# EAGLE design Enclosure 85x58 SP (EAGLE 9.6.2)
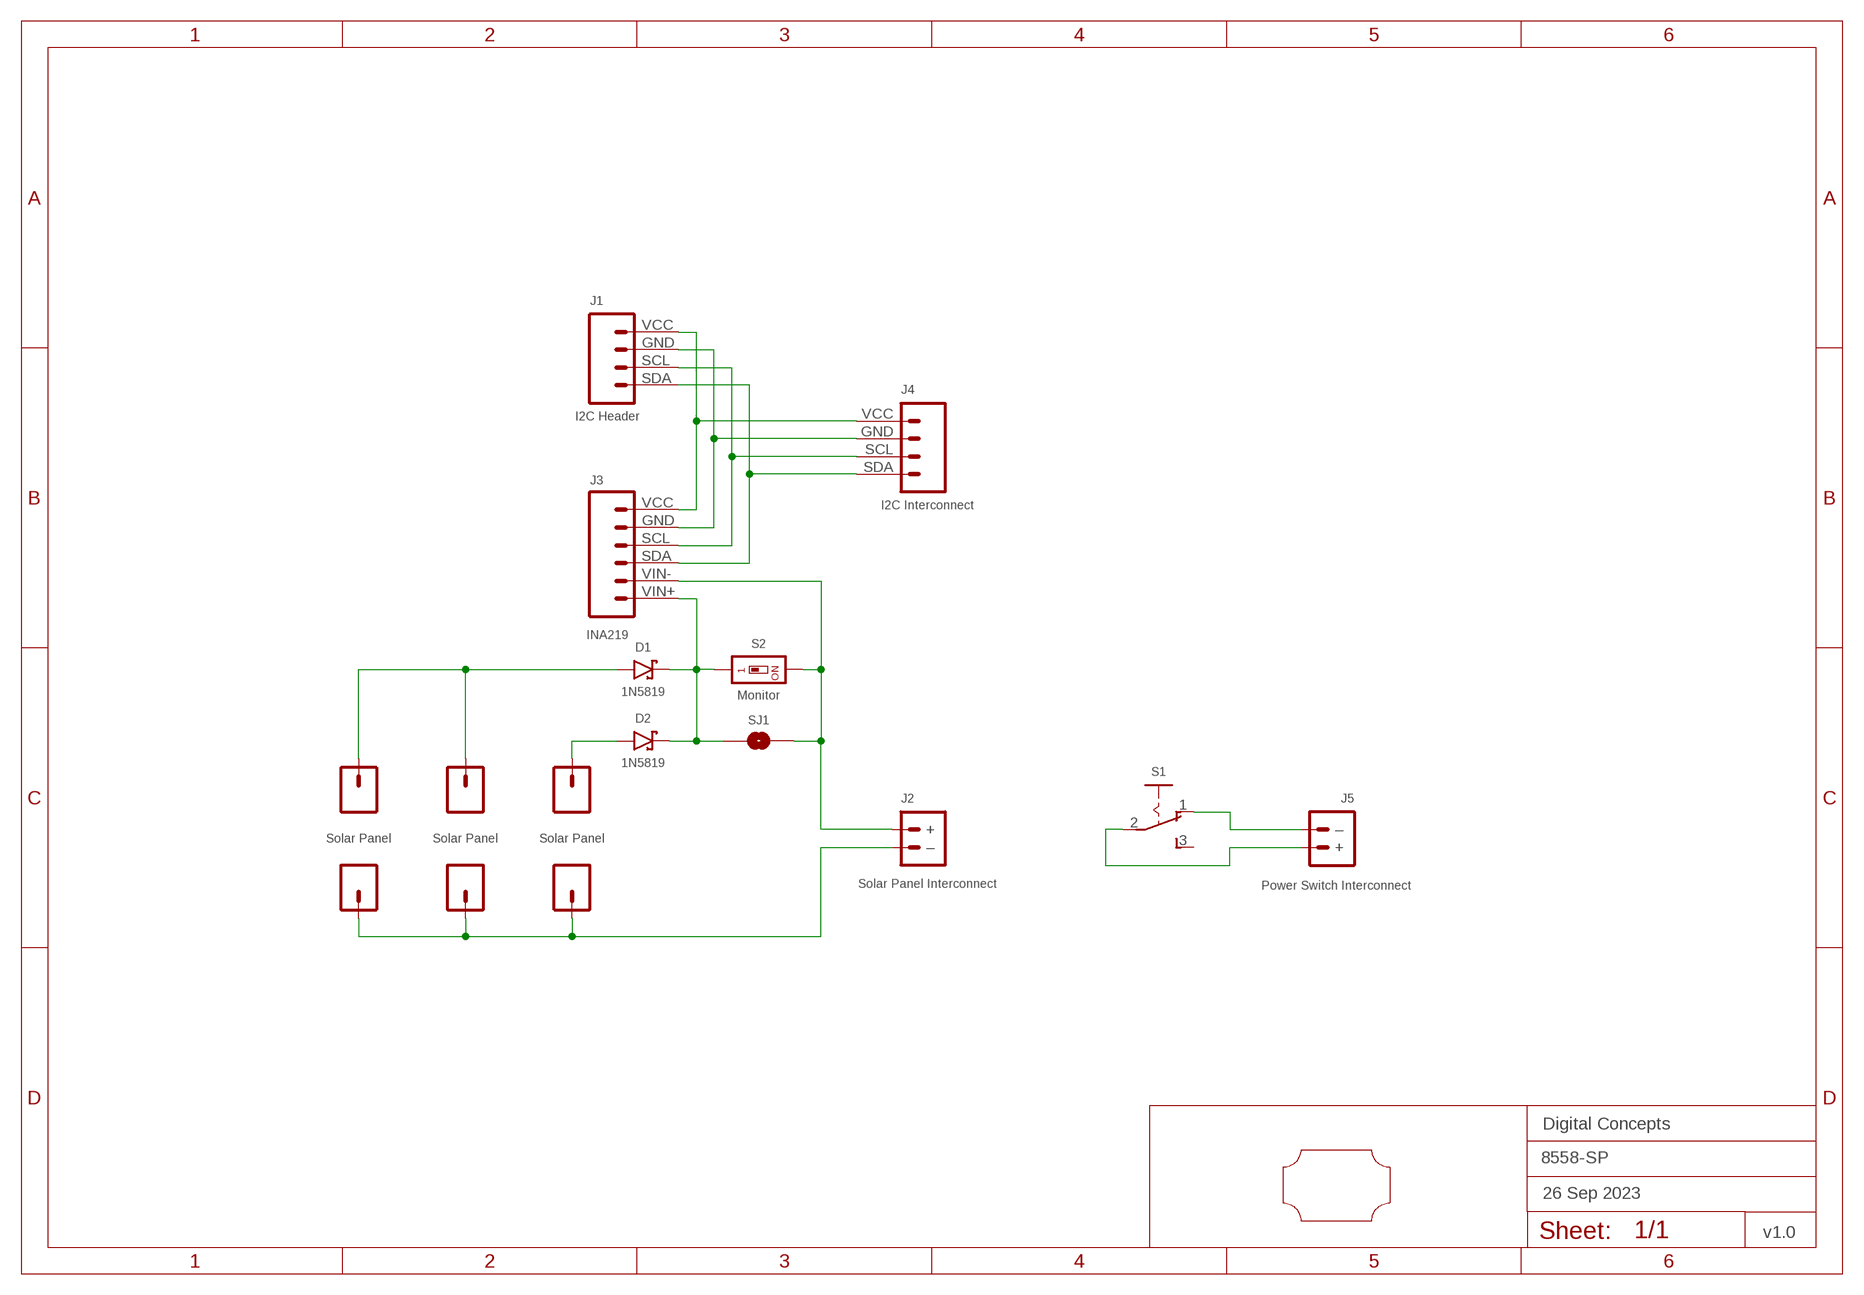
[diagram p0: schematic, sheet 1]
FRAME2 (FRAME-A4L-LOC): DATE: 26 Sep 2023; OWNER: Digital Concepts; TITLE: 8558-SP; VERSION: v1.0

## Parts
+  Solar Panel  PAD-SMD-GENERIC-SQUARE  [PAD-SMD-GENERIC]
+1  Solar Panel  PAD-SMD-GENERIC-SQUARE  [PAD-SMD-GENERIC]
+2  Solar Panel  PAD-SMD-GENERIC-SQUARE  [PAD-SMD-GENERIC]
-  Solar Panel  PAD-SMD-GENERIC-SQUARE  [PAD-SMD-GENERIC]
-1  Solar Panel  PAD-SMD-GENERIC-SQUARE  [PAD-SMD-GENERIC]
-2  Solar Panel  PAD-SMD-GENERIC-SQUARE  [PAD-SMD-GENERIC]
D1  1N5819  DIODE-SCHOTTKY-1N5819  [SOD-123]
D2  1N5819  DIODE-SCHOTTKY-1N5819  [SOD-123]
J1  I2C Header  HEADER-1X4-I2C  [CONN_04-I2C]
J2  Solar Panel Interconnect  JST-PH2.0-2-HORIZONTALJST-PTH-2  [JST-PH2.0-2-HORIZONTAL]
J3  INA219  INA219-I2C-MODULE  [CONN_06-INA219]
J4  I2C Interconnect  JST-PH2.0-4-I2C-HORIZONTAL  [JST-PH2.0-4-HORIZONTAL]
J5  Power Switch Interconnect  JST-PH2.0-2-HORIZONTALJST-PTH-2  [JST-PH2.0-2-HORIZONTAL]
S1  SWITCH-SLIDE-SPDT  [SWITCH-SPDT-PTH]
S2  Monitor  SWITCH-DIP-SWS001  [SMD-001]
SJ1  SJ  [SJ]
U$1  PROTO-28X18-SP  [PROTO-28X18-SP]

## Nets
GND: J1.GND J3.GND J4.GND
N$1: J1.SDA J3.SDA J4.SDA
N$2: J1.SCL J3.SCL J4.SCL
N$3: -1.P$1 -2.P$1 -.P$1 J2.2(–)
N$4: J2.1(+) J3.VIN- S2.2 SJ1.2
N$5: D1.C D2.C J3.VIN+ S2.1 SJ1.1
N$6: J5.1(+) S1.2(P)
N$7: +1.P$1 +2.P$1 D1.A
N$8: +.P$1 D2.A
N$9: J5.2(–) S1.1(O)
VCC: J1.VCC J3.VCC J4.VCC
Unconnected: S1.3(S)

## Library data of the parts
+ +1 +2 - -1 -2 = digitalconcepts:PAD-SMD-GENERIC-SQUARE: SMD Pad—Square
D1 D2 = digitalconcepts:DIODE-SCHOTTKY-1N5819: 1N5819 Schottky Diode SOD-123
J1 = digitalconcepts:HEADER-1X4-I2C: I2C Interface [Pin 1 Vcc] 4-Pin Header
J2 J5 = digitalconcepts:JST-PH2.0-2-HORIZONTAL: PH2.0 2P Right Angle PCB Connector; PROD_ID: CONN-09863; SKU: PRT-09914
J3 = digitalconcepts:INA219-I2C-MODULE: INA219 I2C Module
J4 = digitalconcepts:JST-PH2.0-4-I2C-HORIZONTAL: PH2.0 4P I2C Horizontal Connector
S1 = digitalconcepts:SWITCH-SLIDE-SPDT: Mini Sliding Switch SPDT
S2 = digitalconcepts:SWITCH-DIP-SWS001: SMD Dip Switch 1 pol.
SJ1 = digitalconcepts:SJ: Solder Jumper
U$1 = digitalconcepts:PROTO-28X18-SP: 28 x 18 Prototyping board to fit an 85 x 58 enclosure—Solar panel support

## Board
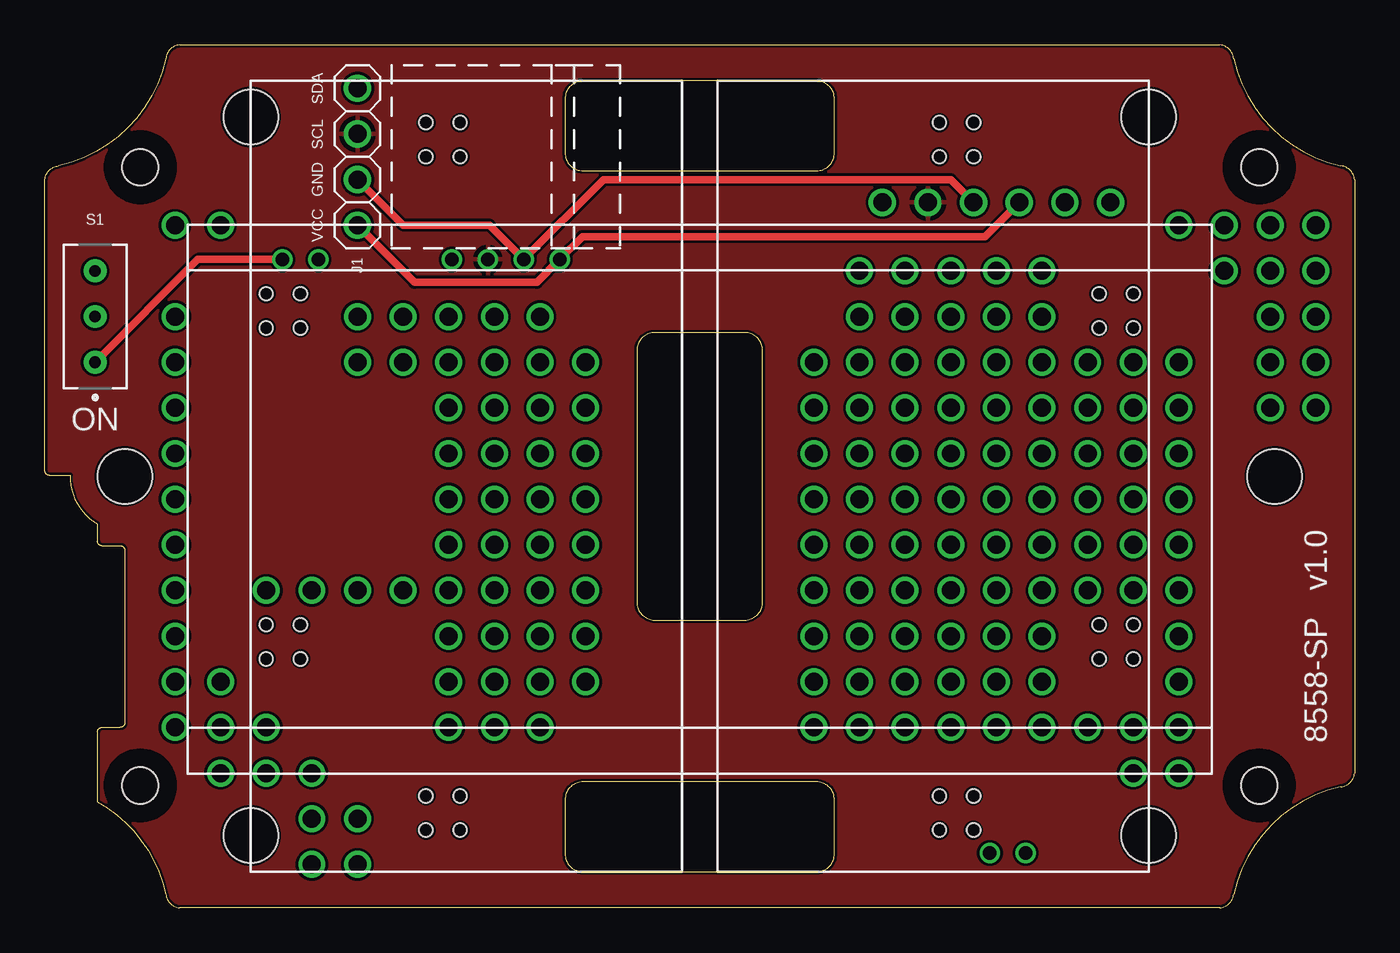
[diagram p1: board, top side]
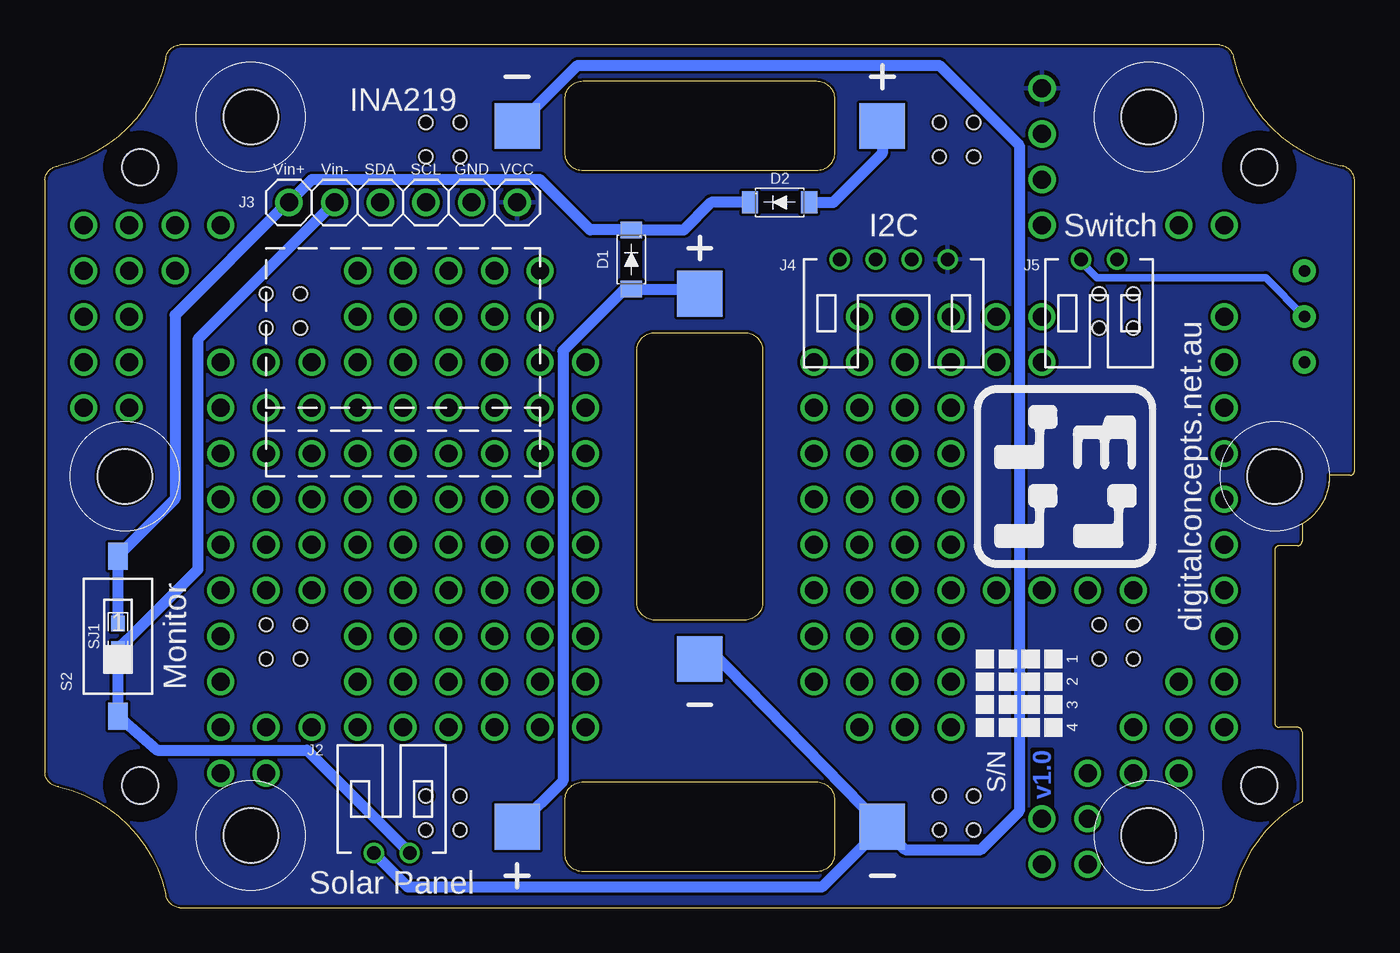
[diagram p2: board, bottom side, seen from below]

Size 72.9 x 48.01 mm. Coordinates in mm from the lower left corner, seen from the top.
Copper layers (1*16): Top 0.035mm / dielectric 1.5mm / Bottom 0.035mm
Design rules "default *": minimum track width 6mil, minimum drill 0.35mm, track to track 6mil, track to pad 6mil, pad to pad 6mil, via to via 6mil, smd to smd 6mil, copper to edge 6mil, drill to drill 6mil, minimum pad ring 1mil, minimum via ring 8mil, stop-mask expansion 4mil, vias tented up to drill 0mil, thermal gap 10mil

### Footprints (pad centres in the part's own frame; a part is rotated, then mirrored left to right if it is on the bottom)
PAD-SMD-GENERIC = smd 2.54 x 2.54: P$1 0,0
SOD-123 = smd 0.91 x 1.22: A -1.65,0; C 1.65,0
CONN_04-I2C = drill 1 pad 1.524: GND 2.54,0; SCL 5.08,0; SDA 7.62,0; VCC 0,0
JST-PH2.0-2-HORIZONTAL = drill 0.75: 1 1,0; 2 -1,0
CONN_06-INA219 = drill 1 pad 1.524: GND 2.54,0; SCL 5.08,0; SDA 7.62,0; VCC 0,0; VIN+ 12.7,0; VIN- 10.16,0
JST-PH2.0-4-HORIZONTAL = drill 0.75: GND -1,0; SCL 1,0; SDA 3,0; VCC -3,0
SWITCH-SPDT-PTH = drill 0.65 pad 1.27: 1 -2.54,0; 2 0,0; 3 2.54,0
SMD-001 = smd 1.1 x 1.5: 1 0,-4.45; 2 0,4.45
SJ = smd 0.864 x 0.762: 1 -0.711,0; 2 0.711,0
PROTO-28X18-SP = drill 1: P03-04 -29.21,-13.97; P03-05 -29.21,-11.43; P03-06 -29.21,-8.89; P03-07 -29.21,-6.35; P03-08 -29.21,-3.81; P03-09 -29.21,-1.27; P03-10 -29.21,1.27; P03-11 -29.21,3.81; P03-12 -29.21,6.35; P03-13 -29.21,8.89; P03-15 -29.21,13.97; P04-03 -26.67,-16.51; P04-04 -26.67,-13.97; P04-05 -26.67,-11.43; P04-15 -26.67,13.97; P05-03 -24.13,-16.51; P05-04 -24.13,-13.97; P05-07 -24.13,-6.35; P06-01 -21.59,-21.59; P06-02 -21.59,-19.05; P06-03 -21.59,-16.51; P06-07 -21.59,-6.35; P07-01 -19.05,-21.59; P07-02 -19.05,-19.05; P07-07 -19.05,-6.35; P07-12 -19.05,6.35; P07-13 -19.05,8.89; P08-07 -16.51,-6.35; P08-12 -16.51,6.35; P08-13 -16.51,8.89; P09-04 -13.97,-13.97; P09-05 -13.97,-11.43; P09-06 -13.97,-8.89; P09-07 -13.97,-6.35; P09-08 -13.97,-3.81; P09-09 -13.97,-1.27; P09-10 -13.97,1.27; P09-11 -13.97,3.81; P09-12 -13.97,6.35; P09-13 -13.97,8.89; P10-04 -11.43,-13.97; P10-05 -11.43,-11.43; P10-06 -11.43,-8.89; P10-07 -11.43,-6.35; P10-08 -11.43,-3.81; P10-09 -11.43,-1.27; P10-10 -11.43,1.27; P10-11 -11.43,3.81; P10-12 -11.43,6.35; P10-13 -11.43,8.89; P11-04 -8.89,-13.97; P11-05 -8.89,-11.43; P11-06 -8.89,-8.89; P11-07 -8.89,-6.35; P11-08 -8.89,-3.81; P11-09 -8.89,-1.27; P11-10 -8.89,1.27; P11-11 -8.89,3.81; P11-12 -8.89,6.35; P11-13 -8.89,8.89; P12-05 -6.35,-11.43; P12-06 -6.35,-8.89; P12-07 -6.35,-6.35; P12-08 -6.35,-3.81; P12-09 -6.35,-1.27; P12-10 -6.35,1.27; P12-11 -6.35,3.81; P12-12 -6.35,6.35; P17-04 6.35,-13.97; P17-05 6.35,-11.43; P17-06 6.35,-8.89; P17-07 6.35,-6.35; P17-08 6.35,-3.81; P17-09 6.35,-1.27; P17-10 6.35,1.27; P17-11 6.35,3.81; P17-12 6.35,6.35; P18-04 8.89,-13.97; P18-05 8.89,-11.43; P18-06 8.89,-8.89; P18-07 8.89,-6.35; P18-08 8.89,-3.81; P18-09 8.89,-1.27; P18-10 8.89,1.27; P18-11 8.89,3.81; P18-12 8.89,6.35; P18-13 8.89,8.89; P18-14 8.89,11.43; P19-04 11.43,-13.97; P19-05 11.43,-11.43; P19-06 11.43,-8.89; P19-07 11.43,-6.35; P19-08 11.43,-3.81; P19-09 11.43,-1.27; P19-10 11.43,1.27; P19-11 11.43,3.81; P19-12 11.43,6.35; P19-13 11.43,8.89; P19-14 11.43,11.43; P20-04 13.97,-13.97; P20-05 13.97,-11.43; P20-06 13.97,-8.89; P20-07 13.97,-6.35; P20-08 13.97,-3.81; P20-09 13.97,-1.27; P20-10 13.97,1.27; P20-11 13.97,3.81; P20-12 13.97,6.35; P20-13 13.97,8.89; P20-14 13.97,11.43; P21-04 16.51,-13.97; P21-05 16.51,-11.43; P21-06 16.51,-8.89; P21-07 16.51,-6.35; P21-08 16.51,-3.81; P21-09 16.51,-1.27; P21-10 16.51,1.27; P21-11 16.51,3.81; P21-12 16.51,6.35; P21-13 16.51,8.89; P21-14 16.51,11.43; P22-04 19.05,-13.97; P22-05 19.05,-11.43; P22-06 19.05,-8.89; P22-07 19.05,-6.35; P22-08 19.05,-3.81; P22-09 19.05,-1.27; P22-10 19.05,1.27; P22-11 19.05,3.81; P22-12 19.05,6.35; P22-13 19.05,8.89; P22-14 19.05,11.43; P23-04 21.59,-13.97; P23-07 21.59,-6.35; P23-08 21.59,-3.81; P23-09 21.59,-1.27; P23-10 21.59,1.27; P23-11 21.59,3.81; P23-12 21.59,6.35; P24-03 24.13,-16.51; P24-04 24.13,-13.97; P24-07 24.13,-6.35; P24-08 24.13,-3.81; P24-09 24.13,-1.27; P24-10 24.13,1.27; P24-11 24.13,3.81; P24-12 24.13,6.35; P25-03 26.67,-16.51; P25-04 26.67,-13.97; P25-05 26.67,-11.43; P25-06 26.67,-8.89; P25-07 26.67,-6.35; P25-08 26.67,-3.81; P25-09 26.67,-1.27; P25-10 26.67,1.27; P25-11 26.67,3.81; P25-12 26.67,6.35; P25-15 26.67,13.97; P26-14 29.21,11.43; P26-15 29.21,13.97; P27-11 31.75,3.81; P27-12 31.75,6.35; P27-13 31.75,8.89; P27-14 31.75,11.43; P27-15 31.75,13.97; P28-11 34.29,3.81; P28-12 34.29,6.35; P28-13 34.29,8.89; P28-14 34.29,11.43; P28-15 34.29,13.97 | hole 2.032: -31.14,17.196; -31.14,-17.196; 31.14,-17.196; 31.14,17.196 | hole 3.048: -24.994,19.99; -32.004,0; -24.994,-19.99; 24.994,-19.99; 32.004,0; 24.994,19.99 | hole 0.75: -15.24,19.685; -13.335,19.685; -13.335,17.78; -15.24,17.78; 13.335,19.685; 15.24,19.685; 15.24,17.78; 13.335,17.78; 13.335,-17.78; 15.24,-17.78; 15.24,-19.685; 13.335,-19.685; -15.24,-17.78; -13.335,-17.78; -13.335,-19.685; -15.24,-19.685; -24.13,10.16; -22.225,10.16; -22.225,8.255; -24.13,8.255; 22.225,10.16; 24.13,10.16; 24.13,8.255; 22.225,8.255; 22.225,-8.255; 24.13,-8.255; 24.13,-10.16; 22.225,-10.16; -24.13,-8.255; -22.225,-8.255; -22.225,-10.16; -24.13,-10.16

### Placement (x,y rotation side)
+  26.29,43.5 0 bottom
+1  46.61,4.5 0 bottom
+2  36.45,34.16 0 bottom
-  46.61,43.5 0 bottom
-1  26.29,4.5 0 bottom
-2  36.45,13.84 0 bottom
D1  40.26,36.07 90 bottom
D2  32,39.24 180 bottom
J1  17.4,45.59 270 top
J2  53.59,3.05 0 bottom
J3  46.61,39.24 180 bottom
J4  25.65,36.07 180 bottom
J5  14.22,36.07 180 bottom
S1  2.79,32.89 90 top
S2  68.83,15.11 180 bottom
SJ1  68.83,15.11 270 bottom
U$1  36.45,24 0 top

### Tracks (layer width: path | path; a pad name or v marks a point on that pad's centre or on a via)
$X0
  cutout Bottom: 5.31,43.23 arc180 5.31,39.17 arc180
$X1
  cutout Bottom: 67.59,43.23 arc180 67.59,39.17 arc180
$X2
  cutout Bottom: 67.59,8.84 arc180 67.59,4.78 arc180
$X3
  cutout Bottom: 5.31,8.84 arc180 5.31,4.78 arc180
$X4
  cutout Top: 5.31,43.23 arc180 5.31,39.17 arc180
$X5
  cutout Top: 67.59,43.23 arc180 67.59,39.17 arc180
$X6
  cutout Top: 67.59,8.84 arc180 67.59,4.78 arc180
$X7
  cutout Top: 5.31,8.84 arc180 5.31,4.78 arc180
GND
  pour Top: -1.65,49.4 74.55,49.4 74.55,-1.4 -1.65,-1.4
N$1
  Top 0.406: J1.SDA 20.57,34.8 27.38,34.8 J4.SDA 29.92,37.34 52.32,37.34 J3.SDA
N$2
  Top 0.406: J1.SCL 19.94,37.97 24.75,37.97 J4.SCL 31.1,40.51 50.42,40.51 J3.SCL
N$3
  Bottom 0.61: -2.P$1 36,14.48 -1.P$1 | -1.P$1 29.65,1.14 52.69,1.14 J2.2 | -.P$1 43.25,46.86 23.11,46.86 18.67,42.42 18.67,5.37 20.8,3.23 25.02,3.23 -1.P$1
N$4
  Bottom 0.61: J2.1 58.31,8.76 66.65,8.76 68.82,10.66 S2.2 SJ1.2 68.3,14.94 68.26,14.94 64.39,18.81 64.39,31.62 J3.VIN-
N$5
  Bottom 0.61: SJ1.1 S2.1 65.66,22.73 65.66,32.97 59.38,39.24 J3.VIN+ 58.04,40.51 45.34,40.51 42.54,37.72 D1.C 37.34,37.72 35.81,39.24 D2.C
N$6
  Bottom 0.406: J5.1 15.22,35.94 14.33,35.05 4.95,35.05 S1.2
N$7
  Bottom 0.61: +2.P$1 36.83,34.16 37.08,34.42 D1.A 40.64,34.42 44.07,30.99 44.07,7.04 +1.P$1
N$8
  Bottom 0.61: D2.A 29.01,39.24 26.29,41.97 +.P$1
N$9
  Top 0.406: S1.1 8.51,36.07 J5.2
VCC
  pour Bottom (rank 5): -1.02,48.77 73.91,48.77 73.91,-0.76 -1.02,-0.76

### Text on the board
Bottom: v1.0
tPlace: SDA | SCL | GND | VCC | ON | 8558-SP v1.0
bPlace: VCC | GND | SCL | SDA | Vin- | Vin+ | digitalconcepts.net.au | 1 | 2 | 3 | 4 | S/N
bNames: Switch | I2C | Solar Panel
